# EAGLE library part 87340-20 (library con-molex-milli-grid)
RECEPTACAL
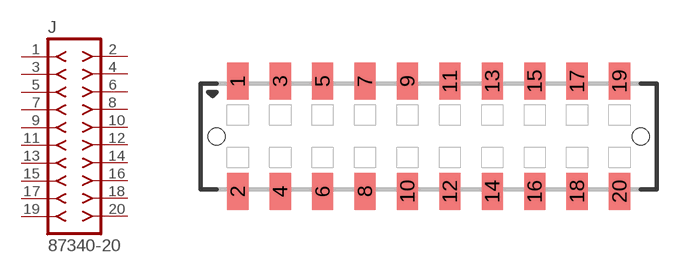
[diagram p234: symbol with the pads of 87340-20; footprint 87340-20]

Designator prefix J

## 87340-20  [87340-20]
1  1  pas
2  2  pas
3  3  pas
4  4  pas
5  5  pas
6  6  pas
7  7  pas
8  8  pas
9  9  pas
10  10  pas
11  11  pas
12  12  pas
13  13  pas
14  14  pas
15  15  pas
16  16  pas
17  17  pas
18  18  pas
19  19  pas
20  20  pas

## Footprint 87340-20 (pad centres in mm)
RECEPTACAL SMD Dual Row, Vertical, Low Profile
smd 1 x 1.75: 1 -9,2.6; 2 -9,-2.6; 3 -7,2.6; 4 -7,-2.6; 5 -5,2.6; 6 -5,-2.6; 7 -3,2.6; 8 -3,-2.6; 9 -1,2.6; 10 -1,-2.6; 11 1,2.6; 12 1,-2.6; 13 3,2.6; 14 3,-2.6; 15 5,2.6; 16 5,-2.6; 17 7,2.6; 18 7,-2.6; 19 9,2.6; 20 9,-2.6
hole 0.8 at -10,0
hole 0.8 at 10,0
